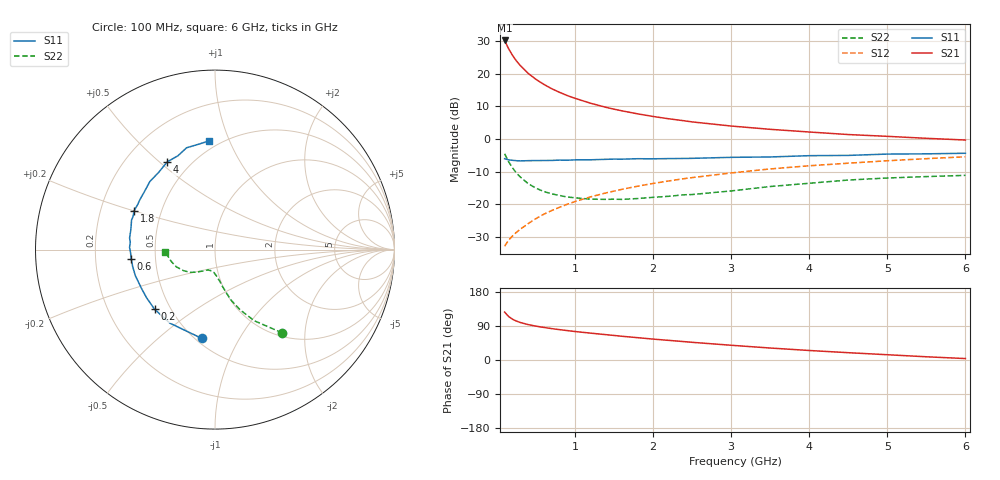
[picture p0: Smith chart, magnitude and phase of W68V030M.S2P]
! SIEMENS Small Signal Semiconductors
! BFR193W
! Si NPN RF Bipolar Junction Transistor in SOT323
! VCE = 8 V  IC = 30 mA
! Common Emitter S-Parameters:  September  1992
# GHz  S  MA  R  50
!  f  S11  S21  S12  S22
! GHz  MAG  ANG  MAG  ANG  MAG  ANG  MAG  ANG
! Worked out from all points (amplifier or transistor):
!   28 points, 100 MHz to 6 GHz, reference 50 ohm
!   highest |S21| = 30.2 dB at 100 MHz (marker M1)
!   |S21| within 3 dB of that: start of sweep to 162.7 MHz
!   unconditionally stable (mu >= 1): 688.8 MHz to 2.605 GHz
!   at 300 MHz: K = 0.83, MSG = 25.1 dB, |S12| = -27.6 dB
!   at 1.5 GHz: K = 1.03, MAG = 11.5 dB, |S12| = -15.9 dB
!   at 6 GHz: K = 0.91, MSG = 2.6 dB, |S12| = -5.4 dB
!   lowest NFmin = 1.90 dB at 450 MHz
!   S11 on the Smith chart (normalised r, x): 100 MHz: 0.54, -0.71; 200 MHz: 0.41, -0.35; 600 MHz: 0.36, -0.05; 1.8 GHz: 0.35, +0.20; 4 GHz: 0.37, +0.53; 6 GHz: 0.44, +0.84
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0.1  0.5003 -98.4  32.37 126.4  0.0229 59.3  0.5961 -51.1
0.15  0.4808 -121.5  24.33 115.0  0.0282 57.9  0.4528 -61.1
0.2  0.473 -135.3  19.23 107.7  0.0327 58.4  0.3644 -67.3
0.25  0.4663 -144.6  15.79 102.8  0.0372 60.0  0.3023 -71.8
0.3  0.4632 -151.7  13.38 99.0  0.0416 61.8  0.263 -74.3
0.4  0.4669 -161.8  10.19 93.5  0.0506 64.5  0.2086 -78.6
0.5  0.4684 -168.2  8.235 89.4  0.0604 66.7  0.1771 -81.6
0.6  0.4695 -173.6  6.906 86.0  0.0705 67.8  0.1578 -85.0
0.7  0.4706 -177.7  5.925 82.9  0.0801 68.7  0.145 -87.2
0.8  0.4762 178.5  5.219 80.2  0.0899 69.2  0.1371 -89.8
0.9  0.4738 175.1  4.648 77.7  0.1002 69.2  0.1296 -91.8
1  0.4804 172.2  4.216 75.2  0.1103 69.3  0.1262 -93.8
1.2  0.4816 166.9  3.539 70.9  0.1302 68.9  0.1201 -99.3
1.5  0.4932 160.6  2.871 64.8  0.1596 67.6  0.12 -105.9
1.8  0.5001 154.3  2.437 59.0  0.1895 66.0  0.1228 -111.6
2.2  0.5021 146.6  2.046 51.8  0.2282 63.3  0.1329 -117.4
3  0.525 133.7  1.584 38.9  0.3028 57.2  0.1606 -128.7
3.5  0.532 126.4  1.41 31.6  0.3487 53.0  0.1876 -137.5
4  0.5567 118.5  1.283 25.1  0.39 48.7  0.2104 -145.9
4.5  0.5619 111.6  1.173 19.3  0.4271 44.6  0.2359 -156.0
5.5  0.594 99.0  1.027 8.5  0.501 36.6  0.2664 -172.9
6  0.6063 93.2  0.967 3.8  0.5358 32.4  0.2781 -177.4
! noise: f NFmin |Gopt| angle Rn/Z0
0.45  1.9  0.4  180  0.09
0.9  1.95  0.43  -173  0.11
1.8  2.4  0.58  -144  0.24
